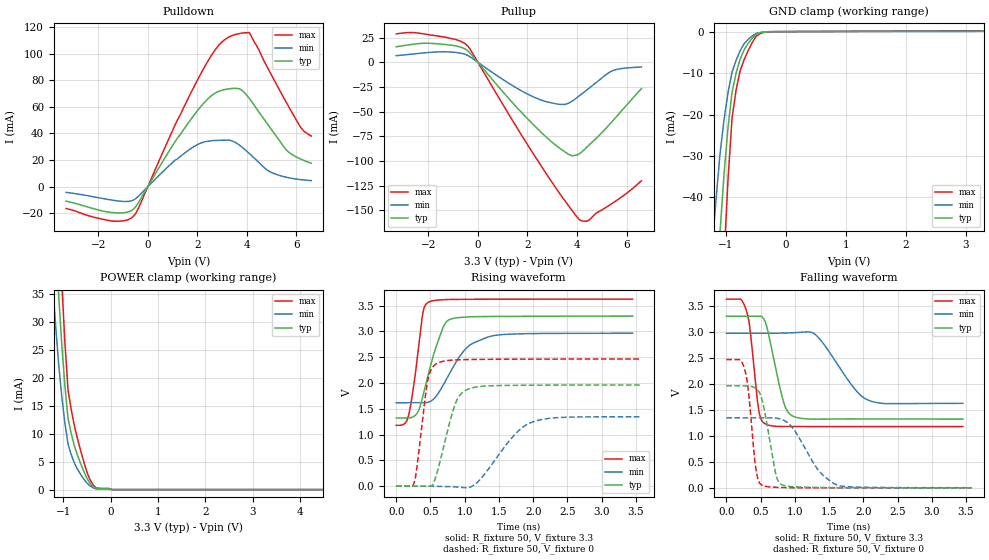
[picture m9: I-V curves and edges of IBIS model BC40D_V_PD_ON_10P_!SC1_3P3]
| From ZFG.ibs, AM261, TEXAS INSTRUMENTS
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[Model]   BC40D_V_PD_ON_10P_!SC1_3P3
Model_type   I/O
Polarity   Non-Inverting
Enable   Active-Low
Vinl =  0.8V
Vinh =  2V
Cref =  15pF
Rref =  100.0000M
Vref =  0V
Vmeas =  1.65
C_comp   2.059994p   1.912853p   2.135747p
|[Input load] weak_pd_on
|[Output drive] fast
|[supplytol] 10
|[temp] ind
[Model Spec]
Vinl   0.8V   0.8V   0.8V
Vinh   2V   2V   2V
[Temperature Range]   25   125   -40
[Voltage Range]   3.3   2.97   3.63
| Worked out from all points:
|   slope of the pulldown table from 0 to 0.495 V, typ, clamps not added: 31.8 ohm
|   slope of the pullup table from 0 to 0.495 V, typ, clamps not added: 33.3 ohm
|   GND clamp passes 1 mA (typ) near -0.52 V on its own axis
|   POWER clamp passes 1 mA (typ) near -0.42 V on its own axis
|   rising waveform, R_fixture 50, V_fixture 3.3: 20-80 % time 251ps typ, 385ps min, 142ps max; typ from 1.32 V to 3.3 V
|   rising waveform, R_fixture 50, V_fixture 0: 20-80 % time 232ps typ, 477ps min, 136ps max; typ from 0 V to 1.96 V
|   falling waveform, R_fixture 50, V_fixture 3.3: 20-80 % time 196ps typ, 423ps min, 118ps max; typ from 3.3 V to 1.32 V
|   falling waveform, R_fixture 50, V_fixture 0: 20-80 % time 159ps typ, 381ps min, 106ps max; typ from 1.96 V to 0 V
| Nom Voltages:
|   VDD=1.1001, VDDS=3.3, VDDS18=1.8, ESD_BIASFET=0, VSS=0, VSSS=0
| Min Voltages:
|   VDD=0.99, VDDS=2.97, VDDS18=1.62, ESD_BIASFET=0, VSS=0, VSSS=0
| Max Voltages:
|   VDD=1.21, VDDS=3.63, VDDS18=1.98, ESD_BIASFET=0, VSS=0, VSSS=0
[POWER_clamp]
|   voltage   I(typ)   I(min)   I(max)
-3.3V     446.9mA    419.5mA    603.9mA
-1.233V   56.59mA    37.53mA    80.37mA
-1.167V   45.68mA    29.91mA    65.17mA
-1.1V     35.14mA    22.68mA    50.36mA
-1.033V   26.13mA    16.78mA    37.31mA
-966.7mV  18.67mA    11.95mA    26.46mA
-900mV    12.76mA    8.172mA    17.82mA
-833.3mV  10.07mA    6.29mA     14.35mA
-566.7mV  3.276mA    1.904mA    4.983mA
-366.7mV  519.9uA    307.2uA    792.3uA
33.33mV   0A         0A         0A
6.6V      0A         0A         0A
[Pulldown]
|   voltage   I(typ)   I(min)   I(max)
-3.3V     -10.92mA   -4.307mA   -16.45mA
-1.4V     -19.52mA   -10.22mA   -25.94mA
-600mV    -17.22mA   -10.25mA   -22.66mA
1.1V      33.8mA     19.88mA    46.22mA
2.1V      59.3mA     32.44mA    83.48mA
2.9V      71.86mA    34.84mA    107mA
3.5V      73.95mA    33.66mA    114.2mA
4.1V      66.34mA    24.89mA    115.8mA
4.9V      45.33mA    11.53mA    87.2mA
5.6V      27.47mA    7.046mA    63.1mA
6.2V      20.56mA    5.221mA    43.87mA
6.6V      17.6mA     4.555mA    38.05mA
[Pullup]
|   voltage   I(typ)   I(min)   I(max)
-3.3V     15.77mA    6.741mA    28.8mA
-1.9V     19.23mA    10.15mA    27.67mA
-900mV    16.69mA    10.02mA    23.17mA
-400mV    11.53mA    6.853mA    16.25mA
1.3V      -38.16mA   -22.04mA   -54.89mA
2.3V      -64.7mA    -35.66mA   -95.04mA
3.3V      -86.93mA   -42.57mA   -132.8mA
3.8V      -94.64mA   -39.36mA   -150mA
4.1V      -92.53mA   -33.79mA   -159.3mA
4.4V      -85.77mA   -27.94mA   -161mA
5.4V      -60.46mA   -8.849mA   -143.2mA
6.6V      -26.71mA   -4.741mA   -120mA
[GND_clamp]
|   voltage   I(typ)   I(min)   I(max)
-3.3V     -787.2mA   -607.8mA   -1.235A
-1.233V   -85.66mA   -52.14mA   -138.8mA
-1.167V   -66.47mA   -40.37mA   -107.7mA
-1.1V     -48.25mA   -29.37mA   -77.99mA
-1.033V   -34.28mA   -21.19mA   -54.56mA
-966.7mV  -23.07mA   -14.67mA   -35.51mA
-900mV    -14.62mA   -9.792mA   -20.84mA
-833.3mV  -10.07mA   -6.938mA   -14.17mA
-700mV    -4.435mA   -2.939mA   -6.836mA
-500mV    -641.2uA   -454.5uA   -1.12mA
-300mV    -31.62uA   -32.73uA   -44.27uA
3.3V      108.6uA    159.4uA    198.5uA
[Ramp]
| variable   typ   min   max
dV/dt_f  1.1955291/0.19759124n 0.83566775/0.43944611n  1.4751133/0.11837667n
dV/dt_r  1.1907008/0.23427848n 0.82841557/0.48868592n  1.4893273/0.136982n
R_load = 50
[Rising Waveform]
R_fixture = 50
V_fixture = 3.3
V_fixture_min = 2.97
V_fixture_max = 3.63
|   time   V(typ)   V(min)   V(max)
0s        1.321V     1.616V     1.179V
178.4ps   1.321V     1.616V     1.359V
304.7ps   1.412V     1.616V     2.443V
385.5ps   1.721V     1.616V     3.326V
470.7ps   2.176V     1.629V     3.567V
685.4ps   3.081V     1.957V     3.616V
810.9ps   3.246V     2.26V      3.62V
1.06ns    3.282V     2.718V     3.624V
1.41ns    3.291V     2.915V     3.625V
3.453ns   3.297V     2.965V     3.627V
[Rising Waveform]
R_fixture = 50
V_fixture = 0
V_fixture_min = 0
V_fixture_max = 0
|   time   V(typ)   V(min)   V(max)
0s        0V         0V         0V
261.9ps   0V         0V         65.75mV
296.9ps   0V         0V         308.5mV
461.7ps   0V         0V         2.052V
529.1ps   19.28mV    -3.671mV   2.304V
597.7ps   265.2mV    -5.419mV   2.381V
855ps     1.568V     -14.09mV   2.447V
1.045ns   1.877V     -30.97mV   2.455V
1.973ns   1.957V     1.235V     2.463V
3.581ns   1.962V     1.343V     2.465V
[Falling Waveform]
R_fixture = 50
V_fixture = 3.3
V_fixture_min = 2.97
V_fixture_max = 3.63
|   time   V(typ)   V(min)   V(max)
0s        3.298V     2.97V      3.626V
295.6ps   3.298V     2.97V      3.395V
344ps     3.298V     2.97V      3.07V
474ps     3.298V     2.97V      1.491V
571.3ps   3.178V     2.97V      1.228V
832.9ps   1.662V     2.974V     1.179V
967ps     1.381V     2.979V     1.179V
1.312ns   1.32V      2.931V     1.179V
2.078ns   1.323V     1.682V     1.178V
3.453ns   1.321V     1.624V     1.178V
[Falling Waveform]
R_fixture = 50
V_fixture = 0
V_fixture_min = 0
V_fixture_max = 0
|   time   V(typ)   V(min)   V(max)
0s        1.961V     1.346V     2.465V
271.4ps   1.96V      1.346V     2.261V
320.4ps   1.959V     1.346V     1.886V
429.7ps   1.91V      1.346V     377.5mV
517.2ps   1.713V     1.346V     52.68mV
725.2ps   253.4mV    1.342V     10.63mV
820.1ps   54.59mV    1.309V     6.154mV
1.353ns   7.192mV    326mV      0V
1.618ns   4.755mV    54.85mV    0V
3.581ns   0V         2.697mV    0V
